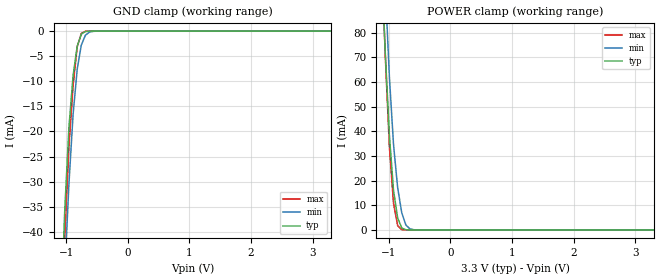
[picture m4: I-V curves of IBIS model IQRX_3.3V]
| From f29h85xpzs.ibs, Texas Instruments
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|IQRX_3.3V;
|   Model IQRX_3.3V
[Model]   IQRX_3.3V
Model_type   Input
Polarity   Non-Inverting
Enable   Active-High
Vinl =   0.800V
Vinh =   2.000V
|   typ   min   max
C_comp   0.537pF   0.535pF   0.543pF
[Model Spec]
Vinh   2.000V   2.000V   2.000V
Vinl   0.800V   0.800V   0.800V
[Temperature Range]   25   155   -40
[Voltage Range]   3.300V   2.800V   3.630V
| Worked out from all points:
|   GND clamp passes 1 mA (typ) near -0.76 V on its own axis
|   POWER clamp passes 1 mA (typ) near -0.79 V on its own axis
[GND_clamp]
|Voltage   I(typ)   I(min)   I(max)
-3.3V     -1.011A    -904.2mA   -1.263A
-1.089V   -56.97mA   -68.01mA   -67.06mA
-1.022V   -35.54mA   -48.03mA   -41.1mA
-955mV    -19.2mA    -30.49mA   -22.97mA
-888mV    -8.936mA   -16.69mA   -10.94mA
-821mV    -3.034mA   -7.611mA   -3.152mA
-754mV    -618.9uA   -2.783mA   -474.6uA
-687mV    -85.76uA   -805.6uA   -42.99uA
-620mV    -11.11uA   -197.4uA   -6.528uA
-486mV    -598.2nA   -9.616uA   -1.017uA
3.3V      0A         0A         0A
[POWER_clamp]
|Voltage   I(typ)   I(min)   I(max)
-3.3V     1.743A     2.034A     1.834A
-1.122V   112.2mA    143.1mA    114.9mA
-1.055V   71.99mA    99.15mA    70.8mA
-988mV    38.41mA    62.04mA    33.74mA
-921mV    16.05mA    34.6mA     10.78mA
-854mV    4.872mA    17.14mA    1.783mA
-787mV    781.4uA    6.912mA    112.7uA
-720mV    79.05uA    1.974mA    7.683uA
-653mV    8.172uA    424.4uA    1.714uA
-586mV    1.25uA     81.64uA    672nA
3.3V      0A         0A         0A
